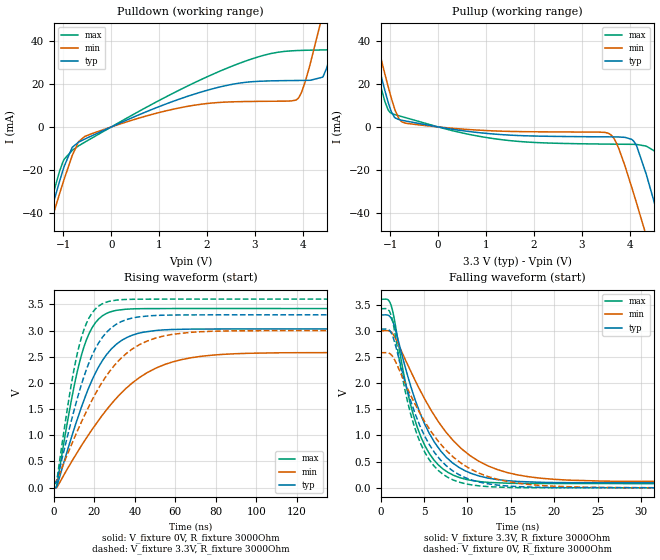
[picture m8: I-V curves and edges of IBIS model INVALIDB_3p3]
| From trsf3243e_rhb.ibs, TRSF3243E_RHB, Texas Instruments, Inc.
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[Model]   INVALIDB_3p3
Model_type   Output
Polarity   Inverting
Vmeas = 2.5
Vref = 2.5
Cref = 30pF
Rref = 0
|   typ   min   max
C_comp   1.21pF   1.18pF   1.21pF
|C_pullup   1.24pF   1.15pF   1.31pF
|C_pulldown   1.68pF   1.64pF   1.74pF
[Voltage Range]   3.3   3   3.6
[Temperature Range]   27   110   -40
[Pullup Reference]   3.3   3   3.6
[Pulldown Reference]   0   0   0
[Power Clamp Reference]   3.3   3   3.6
[GND Clamp Reference]   0   0   0
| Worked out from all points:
|   slope of the pulldown table from 0 to 0.495 V, typ, clamps not added: 101 ohm
|   slope of the pullup table from 0 to 0.495 V, typ, clamps not added: 293 ohm
|   falling waveform, V_fixture 3.3V, R_fixture 3000Ohm: 20-80 % time 4.51ns typ, 6.8ns min, 3.26ns max; typ from 3.3 V to 0.095 V
|   rising waveform, V_fixture 0V, R_fixture 3000Ohm: 20-80 % time 18ns typ, 31.9ns min, 11.1ns max; typ from 0 V to 3.03 V
|   rising waveform, V_fixture 3.3V, R_fixture 3000Ohm: 20-80 % time 15.4ns typ, 24.7ns min, 9.97ns max; typ from 0.095 V to 3.3 V
|   falling waveform, V_fixture 0V, R_fixture 3000Ohm: 20-80 % time 4.36ns typ, 6.28ns min, 3.22ns max; typ from 3.03 V to 0 V
[Pulldown]
|   Voltage   I(typ)   I(min)   I(max)
-3.3V     -210.9mA   -202.6mA   -219.5mA
-1.528V   -61.25mA   -64.54mA   -58.33mA
-1.33V    -45.04mA   -49.56mA   -40.97mA
-983.4mV  -18.34mA   -24.28mA   -15.05mA
-815.1mV  -9.487mA   -13.27mA   -10.92mA
-547.8mV  -5.593mA   -4.392mA   -7.025mA
1.987V    17mA       10.89mA    23.24mA
3.858V    21.65mA    12.57mA    35.59mA
4.412V    23.21mA    52.52mA    35.89mA
4.867V    59.53mA    95.65mA    36.51mA
5.155V    86.82mA    123.4mA    53.5mA
6.6V      228.3mA    265.2mA    193.5mA
[Pullup]
|   Voltage   I(typ)   I(min)   I(max)
-3.3V     228.1mA    235.5mA    222.9mA
-1.865V   87.16mA    95mA       81.48mA
-1.369V   39.85mA    47.85mA    34.03mA
-1.043V   11.33mA    18.58mA    7.778mA
-815.1mV  3.381mA    3.615mA    5.138mA
-676.5mV  2.747mA    1.73mA     4.271mA
3.571V    -4.605mA   -3.149mA   -7.965mA
4.085V    -6.702mA   -31.23mA   -8.08mA
4.343V    -21.86mA   -50.37mA   -8.884mA
4.61V     -42.95mA   -70.75mA   -15.04mA
5.006V    -75.67mA   -101.4mA   -47.2mA
6.6V      -210.8mA   -226.5mA   -191.7mA
[Ramp]
R_load = 3000
|   typ   min   max
dV/dt_r   1.8184/1.80412e-08   1.54816/3.18736e-08   2.05209/1.11116e-08
dV/dt_f   1.92312/4.51136e-09   1.72926/6.79913e-09   2.11219/3.26359e-09
[Falling Waveform]
V_fixture = 3.3V
V_fixture_min = 3V
V_fixture_max = 3.6V
R_fixture = 3000Ohm
C_fixture = 0F
|   Time   V(typ)   V(min)   V(max)
0s        3.3V       3V         3.6V
1.19ns    3.244V     2.976V     3.489V
3.427ns   1.96V      2.239V     1.596V
4.653ns   1.381V     1.828V     964.6mV
5.611ns   1.037V     1.539V     653.9mV
8.957ns   396.7mV    804mV      204.3mV
14.82ns   134.3mV    283.4mV    88.04mV
25.66ns   96.19mV    128.7mV    82.13mV
54.58ns   94.86mV    118mV      79.71mV
1us       94.8mV     117.9mV    79.68mV
[Rising Waveform]
V_fixture = 0V
V_fixture_min = 0V
V_fixture_max = 0V
R_fixture = 3000Ohm
C_fixture = 0F
|   Time   V(typ)   V(min)   V(max)
0s        -282.5nV   -272.4nV   -183.7nV
1.489ns   25.7mV     6.253mV    54.07mV
9.826ns   1.099V     563mV      1.898V
16.07ns   1.793V     946.5mV    2.82V
23.93ns   2.424V     1.382V     3.28V
35.38ns   2.853V     1.885V     3.407V
46.09ns   2.979V     2.196V     3.419V
58.82ns   3.02V      2.403V     3.42V
96.3ns    3.031V     2.566V     3.42V
1us       3.031V     2.58V      3.42V
[Rising Waveform]
V_fixture = 3.3V
V_fixture_min = 3V
V_fixture_max = 3.6V
R_fixture = 3000Ohm
C_fixture = 0F
|   Time   V(typ)   V(min)   V(max)
0s        94.8mV     117.9mV    79.68mV
1.489ns   132mV      137.8mV    145.3mV
9.082ns   1.343V     854mV      2.072V
11.55ns   1.698V     1.076V     2.555V
14.82ns   2.113V     1.353V     3.012V
20.54ns   2.655V     1.792V     3.414V
31.07ns   3.125V     2.384V     3.582V
50.27ns   3.288V     2.857V     3.6V
89.62ns   3.3V       2.995V     3.6V
1us       3.3V       3V         3.6V
[Falling Waveform]
|Gnd
V_fixture = 0V
V_fixture_min = 0V
V_fixture_max = 0V
R_fixture = 3000Ohm
C_fixture = 0F
|   Time   V(typ)   V(min)   V(max)
0s        3.031V     2.58V      3.42V
1.19ns    2.965V     2.545V     3.299V
2.502ns   2.205V     2.114V     2.114V
3.427ns   1.678V     1.778V     1.425V
4.653ns   1.137V     1.386V     825.7mV
5.611ns   824.1mV    1.125V     533.3mV
8.957ns   257.8mV    511mV      114.6mV
14.82ns   33.1mV     116.1mV    7.695mV
32.92ns   2.382mV    1.46mV     604.5uV
1us       -199.9nV   -235.8nV   -264.5nV
